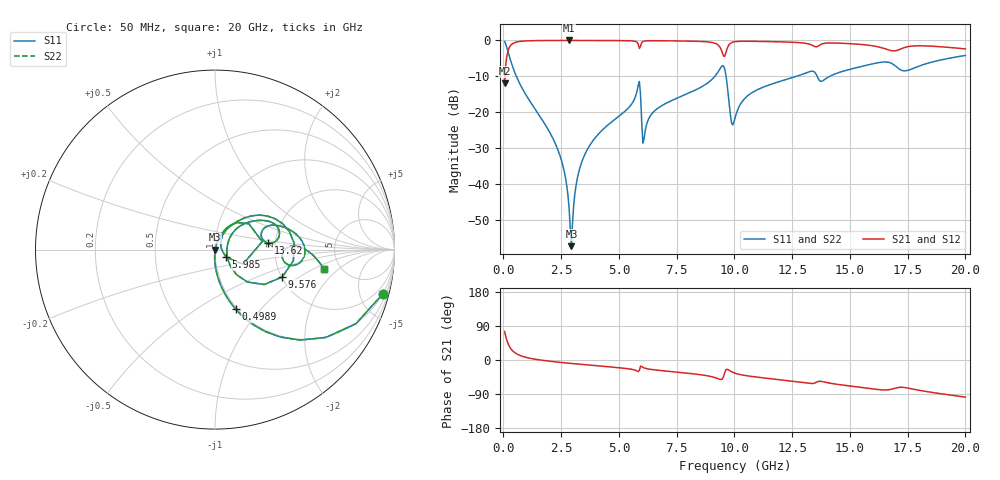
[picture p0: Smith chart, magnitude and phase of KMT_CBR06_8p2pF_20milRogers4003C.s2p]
! Data measured by Modelithics Inc. support@modelithics.com 813-866-6335
! KEMET CBR0603 8.2pF, Pad Width= 0.851mm, Pad Length= 0.64mm, Pad Gap= 0.62mm, 20mil Rogers 4003C substrate Data, January 2022
# hz S ma R 50
! 2 Port Network Data from SP1.SP block
! freq  magS11  angS11  magS21  angS21  magS12  angS12  magS22  angS22
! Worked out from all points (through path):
!   401 points, 50 MHz to 20 GHz, reference 50 ohm
!   highest |S21| = -0.01 dB at 2.843 GHz (marker M1); lowest = -12.0 dB at 50 MHz (marker M2)
!   group delay of S21, straight-line fit = 14.6 ps
!   lowest |S11| = -57.4 dB at 2.943 GHz (marker M3), VSWR 1.00, Z = 50.1 + j0.0126 ohm
!   |S11| at or under -10 dB: 557.4 MHz to 9.154 GHz (8.596 GHz wide, 177 % of centre); 9.637 GHz to 12.69 GHz (3.057 GHz wide, 27.4 % of centre); 13.58 GHz to 14.13 GHz (548.2 MHz wide, 3.96 % of centre)
!   |S22| runs from -57.4 to -0.3 dB; largest |S21 - S12| = 0
!   S11 on the Smith chart (normalised r, x): 50 MHz: 0.98, -7.62; 498.9 MHz: 0.98, -0.74; 5.985 GHz: 1.13, -0.10; 9.576 GHz: 2.02, -0.74; 13.62 GHz: 1.84, +0.14; 20 GHz: 3.72, -1.33
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5e7  0.9678 -14.7  0.2513 75.3  0.2513 75.3  0.9678 -14.7
2.495e8  0.6079 -53.2  0.793 36.7  0.793 36.7  0.6079 -53.2
4.98875e8  0.3511 -70.8  0.9354 19.0  0.9354 19.0  0.3511 -70.8
2.34425e9  0.0305 -93.3  0.9983 -5.5  0.9983 -5.5  0.0305 -93.3
2.6435e9  0.01427 -92.3  0.9986 -7.3  0.9986 -7.3  0.01427 -92.3
2.843e9  0.004547 -82.1  0.9986 -8.5  0.9986 -8.5  0.004547 -82.1
2.94275e9  0.00135 5.3  0.9986 -9.1  0.9986 -9.1  0.00135 5.3
3.391625e9  0.02016 74.4  0.9983 -11.6  0.9983 -11.6  0.02016 74.4
5.785625e9  0.198 49.5  0.9412 -29.0  0.9412 -29.0  0.198 49.5
5.985125e9  0.07403 -34.8  0.929 -17.1  0.929 -17.1  0.07403 -34.8
6.13475e9  0.05424 53.1  0.9843 -21.8  0.9843 -21.8  0.05424 53.1
6.73325e9  0.1162 61.0  0.9896 -27.3  0.9896 -27.3  0.1162 61.0
9.177125e9  0.3228 36.3  0.9078 -46.7  0.9078 -46.7  0.3228 36.3
9.576125e9  0.4048 -22.2  0.6001 -34.0  0.6001 -34.0  0.4048 -22.2
9.875375e9  0.07065 -19.8  0.9302 -30.9  0.9302 -30.9  0.07065 -19.8
1.0025e10  0.08237 28.3  0.9597 -34.8  0.9597 -34.8  0.08237 28.3
1.077312e10  0.1877 43.4  0.9722 -43.6  0.9722 -43.6  0.1877 43.4
1.336662e10  0.3728 16.7  0.8572 -62.0  0.8572 -62.0  0.3728 16.7
1.3616e10  0.2996 6.7  0.8294 -56.8  0.8294 -56.8  0.2996 6.7
1.670825e10  0.4917 -6.3  0.7309 -78.2  0.7309 -78.2  0.4917 -6.3
1.74065e10  0.3764 -3.7  0.802 -73.0  0.802 -73.0  0.3764 -3.7
2e10  0.6175 -10.3  0.761 -98.0  0.761 -98.0  0.6175 -10.3
